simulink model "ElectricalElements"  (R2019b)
settings: Solver=ode45  StartTime=0.0  StopTime=10.0  RelTol=1e-3  EnableMultiTasking=on

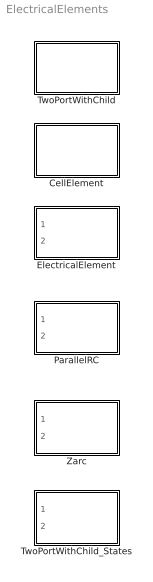
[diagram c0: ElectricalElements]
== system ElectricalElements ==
  CellElement : Subsystem
  ElectricalElement : Subsystem
  ParallelRC : Subsystem
  TwoPortWithChild : Subsystem
  TwoPortWithChild_States : Subsystem
  Zarc : Subsystem

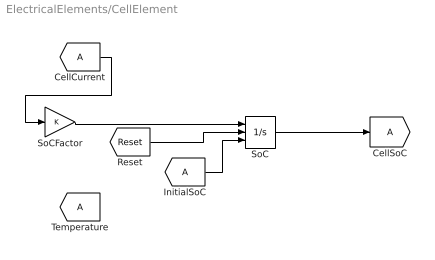
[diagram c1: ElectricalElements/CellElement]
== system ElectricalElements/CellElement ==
  CellCurrent : From  TagVisibility=global
  CellSoC : Goto  TagVisibility=global
  InitialSoC : From  TagVisibility=global
  SoC : Integrator  ExternalReset=rising  InitialConditionSource=external  LimitOutput=on  UpperSaturationLimit=100  LowerSaturationLimit=0
  SoCFactor : Gain
  Temperature : From  TagVisibility=global
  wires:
  SoCFactor/1 -> SoC/1
  CellCurrent/1 -> SoCFactor/1
  SoC/1 -> CellSoC/1
  [Reset] -> SoC/2
  InitialSoC/1 -> SoC/3

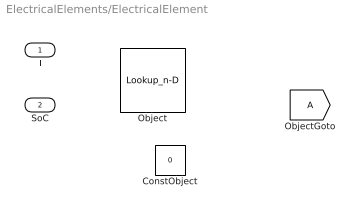
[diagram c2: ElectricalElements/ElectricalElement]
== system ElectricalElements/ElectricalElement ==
  T : Inport
  SoC : Inport  Port=2
  ConstObject : Constant  Value=0
  Object : Lookup_n-D  Table=[1,2,3;4,5,6;7,8,9]  ExtrapMethod=Clip  RndMeth=Simplest
  ObjectGoto : Goto  TagVisibility=global

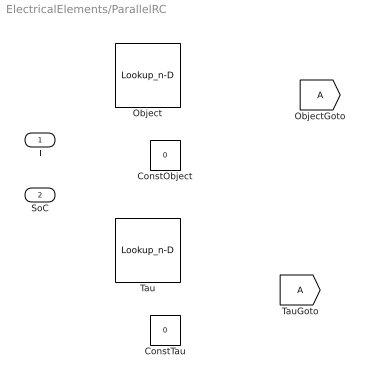
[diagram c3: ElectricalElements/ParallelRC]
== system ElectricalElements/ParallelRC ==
  T : Inport
  SoC : Inport  Port=2
  ConstObject : Constant  Value=0
  ConstTau : Constant  Value=0
  Object : Lookup_n-D  Table=[1,2,3;4,5,6;7,8,9]  ExtrapMethod=Clip  RndMeth=Simplest
  ObjectGoto : Goto  TagVisibility=global
  Tau : Lookup_n-D  Table=[1,2,3;4,5,6;7,8,9]  ExtrapMethod=Clip  RndMeth=Simplest
  TauGoto : Goto  TagVisibility=global

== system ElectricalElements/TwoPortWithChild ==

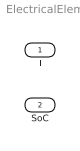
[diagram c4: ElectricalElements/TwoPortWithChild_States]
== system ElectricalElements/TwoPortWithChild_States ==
  T : Inport
  SoC : Inport  Port=2

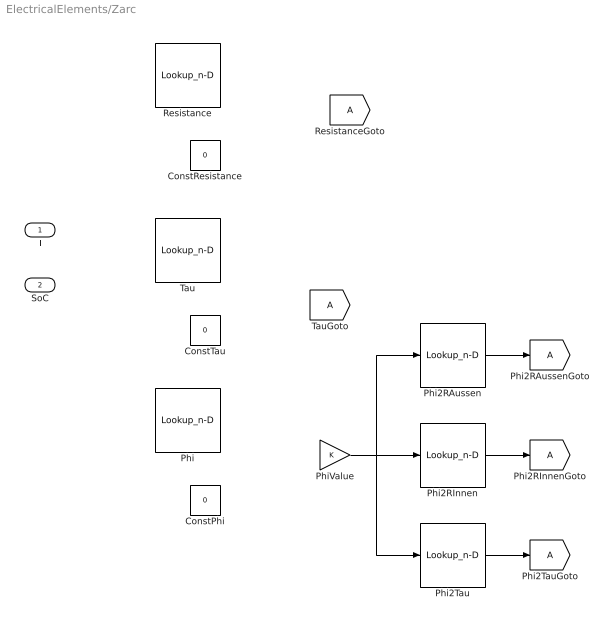
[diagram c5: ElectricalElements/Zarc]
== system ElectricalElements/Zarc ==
  T : Inport
  SoC : Inport  Port=2
  ConstPhi : Constant  Value=0
  ConstResistance : Constant  Value=0
  ConstTau : Constant  Value=0
  Phi : Lookup_n-D  Table=[1,2,3;4,5,6;7,8,9]  ExtrapMethod=Clip  RndMeth=Simplest
  Phi2RAussen : Lookup_n-D  NumberOfTableDimensions=1  BreakpointsForDimension1=[-5:5]  Table=tanh([-5:5])  ExtrapMethod=Clip  RndMeth=Simplest
  Phi2RAussenGoto : Goto  TagVisibility=global
  Phi2RInnen : Lookup_n-D  NumberOfTableDimensions=1  BreakpointsForDimension1=[-5:5]  Table=tanh([-5:5])  ExtrapMethod=Clip  RndMeth=Simplest
  Phi2RInnenGoto : Goto  TagVisibility=global
  Phi2Tau : Lookup_n-D  NumberOfTableDimensions=1  BreakpointsForDimension1=[-5:5]  Table=tanh([-5:5])  ExtrapMethod=Clip  RndMeth=Simplest
  Phi2TauGoto : Goto  TagVisibility=global
  PhiValue : Gain
  Resistance : Lookup_n-D  Table=[1,2,3;4,5,6;7,8,9]  ExtrapMethod=Clip  RndMeth=Simplest
  ResistanceGoto : Goto  TagVisibility=global
  Tau : Lookup_n-D  Table=[1,2,3;4,5,6;7,8,9]  ExtrapMethod=Clip  RndMeth=Simplest
  TauGoto : Goto  TagVisibility=global
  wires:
  Phi2RAussen/1 -> Phi2RAussenGoto/1
  Phi2RInnen/1 -> Phi2RInnenGoto/1
  Phi2Tau/1 -> Phi2TauGoto/1
  PhiValue/1 -> Phi2Tau/1, Phi2RAussen/1, Phi2RInnen/1
